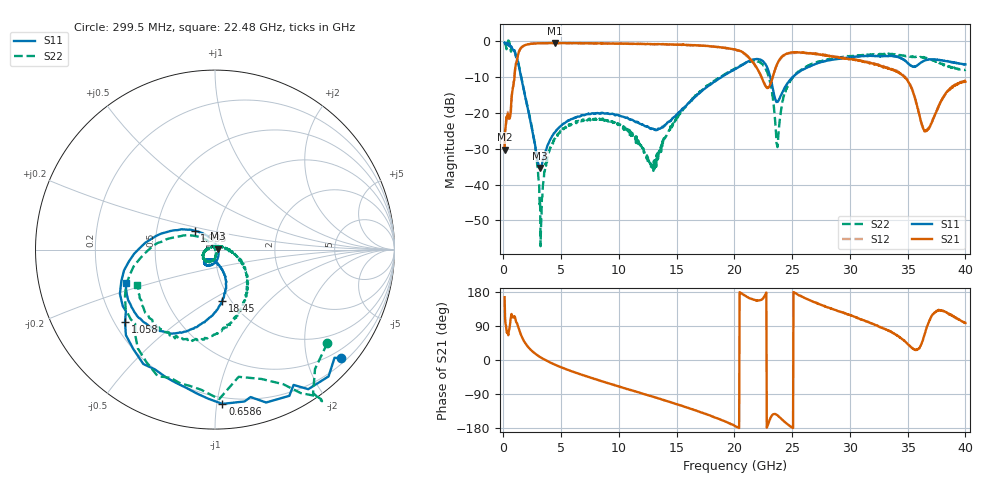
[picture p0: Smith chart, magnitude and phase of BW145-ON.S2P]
!  2-Port S-parameters saved by WinCal
! VAR MeasName=S-Parameters (CALIBRATED_DATA) read from VNA (E8364A)
! VAR MeasDate=5/8/2013 4:32:48 PM
! VAR NAME=131606
! VAR FILENAME=131606.S2P
! VAR DATE=5/8/2013 4:32:48 PM
! VAR PHYS_PORTS=1,2
# Hz S MA R 50
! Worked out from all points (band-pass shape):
!   1001 points, 100 MHz to 40 GHz, reference 50 ohm
!   highest |S21| = -0.43 dB at 4.489 GHz (marker M1); lowest = -30.2 dB at 100 MHz (marker M2)
!   |S21| within 3 dB of the highest: 1.285 GHz to 20.88 GHz (19.6 GHz wide, 177 % of centre); 24.56 GHz to 26.78 GHz (2.216 GHz wide, 8.63 % of centre)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
!   lowest |S11| = -35.3 dB at 3.172 GHz (marker M3), VSWR 1.03, Z = 51.7 + j0.455 ohm
!   |S11| at or under -10 dB: 1.531 GHz to 18.86 GHz (17.33 GHz wide, 170 % of centre); 23.11 GHz to 25.04 GHz (1.925 GHz wide, 8 % of centre)
!   |S22| runs from -57.2 to 0.3 dB; largest |S21 - S12| = 0.034
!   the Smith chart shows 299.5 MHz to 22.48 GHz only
!   S11 on the Smith chart (normalised r, x): 299.5 MHz: 0.30, -2.66; 658.6 MHz: 0.16, -1.04; 1.058 GHz: 0.24, -0.33; 1.935 GHz: 0.78, +0.17; 18.45 GHz: 0.92, -0.57; 22.48 GHz: 0.32, -0.16
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1e8  0.9651 -15.1  0.03088 165.8  0.03081 166.7  0.9686 -14.1
2.995e8  0.9288 -40.7  0.08576 71.8  0.0843 70.0  0.8145 -39.8
6.586e8  0.8606 -87.3  0.1278 114.3  0.1115 115.7  0.7209 -79.5
1.0576e9  0.6443 -141.1  0.4659 105.6  0.464 106.0  0.6492 -133.3
1.4566e9  0.3614 170.7  0.7867 71.2  0.7863 71.2  0.3712 -179.7
1.9354e9  0.1536 136.9  0.8991 42.7  0.8992 42.5  0.1582 149.9
2.7733e9  0.03266 84.6  0.9389 16.4  0.9384 16.3  0.03227 121.2
3.1723e9  0.0171 14.9  0.944 7.9  0.9459 7.9  0.005874 95.2
4.489e9  0.05494 -75.8  0.9519 -12.7  0.9512 -12.8  0.04462 -87.7
6.7633e9  0.09227 -108.3  0.9467 -38.9  0.943 -38.5  0.07771 -119.6
1.34266e10  0.05937 -99.0  0.9172 -101.5  0.9184 -101.6  0.02574 35.9
1.8454e10  0.2873 -81.8  0.8413 -153.3  0.8399 -153.4  0.291 -53.3
2.005e10  0.4102 -98.8  0.7747 -174.4  0.7698 -174.3  0.4148 -77.3
2.24839e10  0.5281 -159.5  0.2801 162.6  0.2844 163.8  0.4767 -155.5
2.31223e10  0.3109 175.0  0.255 -152.7  0.2526 -153.1  0.2503 162.9
2.37208e10  0.143 -149.0  0.492 -146.2  0.4875 -146.0  0.03342 37.5
2.46784e10  0.2716 -117.5  0.6882 -171.2  0.6762 -170.4  0.2577 -58.8
2.67133e10  0.4644 -133.8  0.6777 155.3  0.6845 156.6  0.4899 -99.3
3.33766e10  0.6253 146.4  0.4205 76.4  0.4231 78.3  0.665 176.7
3.50524e10  0.4953 116.3  0.2713 40.8  0.28 40.8  0.6251 149.8
3.65686e10  0.5501 106.4  0.05562 78.4  0.05587 78.1  0.588 116.5
4e10  0.4786 1.5  0.274 97.6  0.2831 99.1  0.4044 -2.7
